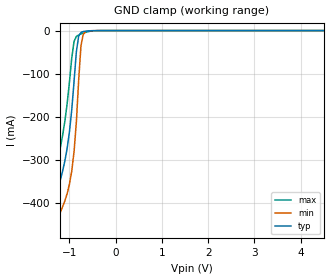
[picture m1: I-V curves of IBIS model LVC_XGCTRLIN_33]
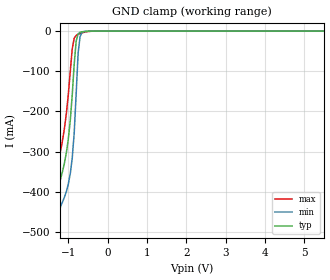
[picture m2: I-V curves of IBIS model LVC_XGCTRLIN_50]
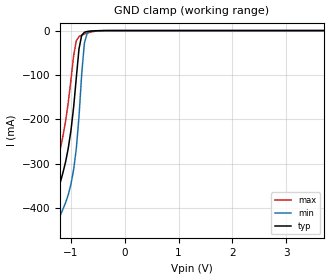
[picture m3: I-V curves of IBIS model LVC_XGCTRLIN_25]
| Philips Semiconductors Inc.
| Logic Products Group
| IBIS model of 74LVC2G125
| 3.3V DUAL BUS BUFFER/LINE DRIVER (3-STATE)
|[Packages]:
|[Package1]: SOT505-2 (TSSOP) 8-Pin Package ;
|[Package2]: SOT765 (VSSOP) 8-Pin Package ;
[IBIS Ver]   3.2
[File Name]   lvc2g125.ibs
[File Rev]   1.0
[Date]   25-Jul-2003
[Source]   File created from simulations by LPG
   Philips Semiconductors Nijmegen
[Notes]   V1.0   Ibis model.
| Revision History
| Version Date   Author/ Description
|   Editor
| 1.0   July   2003 RM   Initial Version
| Remarks:
| 1. The Power Clamp curves have been omitted since there is no power clamp
|   diode.
| 2. Non-monotonic sections below 0V in pulldown and pullup curves have been
|   removed (if any).
[Disclaimer]
   (C) Copyright 2003 Philips Semiconductors
   All rights reserved
   Philips Semiconductors warrants and represents that the IBIS model
   identified herein is owned by Philips Semiconductors (PHILIPS). The
   model provided is not warranted as fully representing all of the
   operating characteristics and specifications of the semiconductor
   products to which the model relates.  Moreover, unless there is a
   signed, written agreement to the contrary, this IBIS model is
   furnished on an "as is" basis without support or warranty of any
   kind, either expressed or implied, regarding the use thereof, and
   PHILIPS specifically disclaims all implied warranties of
   merchantability and fitness of the model for any purpose.
   PHILIPS does not assume any liability arising out of the application
   or use of this IBIS model including infringement of patents and
   copyrights, nor does PHILIPS convey any license under its patents and
   copyrights or the rights of others.
   PHILIPS provides IBIS models as a service to our customers. You and
   your company shall not distribute, convey, sell, or give these models
   to anyone else without receiving prior written permission from
   PHILIPS.
   PHILIPS reserves the right to make changes without notice to these
   IBIS models to improve reliability, function, or design.
   Please be aware that your receipt and subsequent use of the IBIS
   information provided shall serve as acceptance of the terms and
   conditions of this agreement.  If you do not accept these terms,
   you should return or destroy the IBIS models and any other
   accompanying information immediately.
|   Info for  SOT505-2 (TSSOP) 8-Pin Package
[Component]   74LVC2G125_1
[Manufacturer]   Philips Semiconductors Inc.
[Package]
|   typ   min   max
R_pkg   5.4457E-02   4.6527E-02   6.2827E-02
L_pkg   1.399E-09   1.251E-09   1.584E-09
C_pkg   9.08E-14   7.40E-14   1.08E-13
[Pin] signal_name   model_name   R_pin   L_pin   C_pin
   1   OE1#   lvc_xgctrlin 6.28E-02 1.584E-09  1.08E-13
   2   A1   lvc_xgin 4.72E-02 1.312E-09  7.50E-14
   3   Y2   lvc_xgtristn 4.65E-02 1.251E-09  7.40E-14
   4   GND   GND 6.15E-02 1.472E-09  1.07E-13
   5   A2   lvc_xgin 6.22E-02 1.484E-09  1.07E-13
   6   Y1   lvc_xgtristn 4.69E-02 1.256E-09  7.40E-14
   7   OE2#   lvc_xgctrlin 4.67E-02 1.304E-09  7.40E-14
   8   VCC   POWER 6.18E-02 1.527E-09  1.07E-13
|   Info for  SOT765 (VSSOP) 8-Pin Package
[Component]   74LVC2G125_2
[Manufacturer]   Philips Semiconductors Inc.
[Package]
|   typ   min   max
R_pkg   3.2883E-02   1.0000E-06   4.2432E-02
L_pkg   9.425E-10   1.000E-12   1.184E-09
C_pkg   8.64E-14   1.00E-15   1.19E-13
[Pin] signal_name   model_name   R_pin   L_pin   C_pin
   1   OE1#   lvc_xgctrlin 4.24E-02 1.145E-09  1.19E-13
   2   A1   lvc_xgin 3.40E-02 1.018E-09  8.30E-14
   3   Y2   lvc_xgtristn 3.40E-02 1.016E-09  8.40E-14
   4   GND   GND 4.24E-02  1.15E-09  1.19E-13
   5   A2   lvc_xgin 3.40E-02  9.89E-10  1.12E-13
   6   Y1   lvc_xgtristn 3.40E-02 1.037E-09  8.30E-14
   7   OE2#   lvc_xgctrlin 4.24E-02 1.184E-09  9.00E-14
   8   VCC   POWER 1.00E-06  1.00E-12  1.00E-15
[Model Selector]   lvc_xgctrlin
| Remark: If your software does not support the Model Selector
|   Please comment out the lines of the Model Selector, which
|   contain the name of the Model, except the one you want to use.
LVC_XGCTRLIN_33   3.3V-Vcc input model
LVC_XGCTRLIN_50   5.0V-Vcc input model
LVC_XGCTRLIN_25   2.5V-Vcc input model
LVC_XGCTRLIN_18   1.8V-Vcc input model
[Model Selector]   lvc_xgin
| Remark: If your software does not support the Model Selector
|   Please comment out the lines of the Model Selector, which
|   contain the name of the Model, except the one you want to use.
LVC_XGIN_33   3.3V-Vcc input model
LVC_XGIN_50   5.0V-Vcc input model
LVC_XGIN_25   2.5V-Vcc input model
LVC_XGIN_18   1.8V-Vcc input model
[Model Selector]   lvc_xgtristn
| Remark: If your software does not support the Model Selector
|   Please comment out the lines of the Model Selector, which
|   contain the name of the Model, except the one you want to use.
LVC_XGTRISTN_33   3.3V-Vcc tristate non-inverting output model
LVC_XGTRISTN_50   5.0V-Vcc tristate non-inverting output model
LVC_XGTRISTN_25   2.5V-Vcc tristate non-inverting output model
LVC_XGTRISTN_18   1.8V-Vcc tristate non-inverting output model
| Models and submodels in the file (12): LVC_XGCTRLIN_33 (Input), LVC_XGCTRLIN_50 (Input), LVC_XGCTRLIN_25 (Input), LVC_XGCTRLIN_18 (Input), LVC_XGIN_33 (Input), LVC_XGIN_50 (Input), LVC_XGIN_25 (Input), LVC_XGIN_18 (Input), LVC_XGTRISTN_33 (3-state), LVC_XGTRISTN_50 (3-state), LVC_XGTRISTN_25 (3-state), LVC_XGTRISTN_18 (3-state)
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|   Model LVC_XGCTRLIN_33
[Model]   LVC_XGCTRLIN_33
Model_type   Input
Vinl =   0.8V
Vinh =   2.0V
C_comp   2.96pF   2.12pF   3.91pF
[Model Spec]
| Note: The input and output voltage ratings may be exceeded if the input and
|   output current ratings are observed (please refer to the data sheet)
|   Subparameter   typ   min   max
| Thresholds
Vinh   2.0   2.0   2.0
Vinl   0.8   0.8   0.8
| Overshoot
S_overshoot_high   6.5   6.5   6.5   | Static overshoot
S_overshoot_low   -0.5   -0.5   -0.5
D_overshoot_high   7.2   7.2   7.2   | Dynamic overshoot
D_overshoot_low   -0.95   -0.9   -1.0
D_overshoot_time   3n   3n   3n
|Ambient temperature:   25   85   -40
[Temperature Range]   50   105   -10
[Voltage Range]   3.3V   3.0V   3.6V
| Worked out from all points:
|   GND clamp passes 1 mA (typ) near -0.61 V on its own axis
|Process Range   nominal   slow   fast
[GND_clamp]
| voltage   I(typ)   I(min)   I(max)
-5.5V     -4.562A    -4.619A    -4.506A
-1.45V    -549.4mA   -615.4mA   -482.8mA
-1.4V     -502.2mA   -568.5mA   -435.4mA
-1.35V    -455.9mA   -522.5mA   -388.7mA
-1.3V     -411.6mA   -478.9mA   -343.8mA
-1.1V     -304.2mA   -396.4mA   -212.1mA
-950mV    -185.2mA   -327mA     -64.69mA
-850mV    -49.8mA    -213.4mA   -13.79mA
-750mV    -4.324mA   -35.6mA    -7.884mA
-700mV    -2.27mA    -8.526mA   -5.841mA
-550mV    -593.6uA   -425.2uA   -1.597mA
5.5V      375.8pA    2.471nA    52.76pA
|   Model LVC_XGCTRLIN_50
[Model]   LVC_XGCTRLIN_50
Model_type   Input
Vinl =   1.5V
Vinh =   3.5V
C_comp   2.89pF   1.97pF   3.94pF
[Model Spec]
| Note: The input and output voltage ratings may be exceeded if the input and
|   output current ratings are observed (please refer to the data sheet)
|   Subparameter   typ   min   max
| Thresholds
Vinh   3.5   3.15   3.85
Vinl   1.5   1.35   1.65
| Overshoot
S_overshoot_high   6.5   6.5   6.5   | Static overshoot
S_overshoot_low   -0.5   -0.5   -0.5
D_overshoot_high   11.0   11.0   11.0   | Dynamic overshoot
D_overshoot_low   -0.95   -0.9   -1.0
D_overshoot_time   3n   3n   3n
|Ambient temperature:   25   85   -40
[Temperature Range]   50   105   -10
[Voltage Range]   5.0V   4.5V   5.5V
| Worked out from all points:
|   GND clamp passes 1 mA (typ) near -0.59 V on its own axis
|Process Range   nominal   slow   fast
[GND_clamp]
| voltage   I(typ)   I(min)   I(max)
-5.5V     -4.585A    -4.637A    -4.534A
-1.45V    -567.8mA   -628.4mA   -505.9mA
-1.4V     -520.6mA   -581.5mA   -458.5mA
-1.3V     -430.1mA   -491.9mA   -367mA
-1.2V     -369.6mA   -437.9mA   -299.9mA
-1.05V    -303mA     -399.7mA   -205.6mA
-950mV    -222.3mA   -354.8mA   -100.4mA
-850mV    -82.04mA   -253.9mA   -17.37mA
-800mV    -24.94mA   -156mA     -10.72mA
-750mV    -6.792mA   -54.58mA   -8.095mA
-700mV    -2.837mA   -13.44mA   -6.14mA
5.5V      1.794nA    5.479nA    963.8pA
|   Model LVC_XGCTRLIN_25
[Model]   LVC_XGCTRLIN_25
Model_type   Input
Vinl =   0.7V
Vinh =   1.7V
C_comp   3.01pF   2.23pF   3.90pF
[Model Spec]
| Note: The input and output voltage ratings may be exceeded if the input and
|   output current ratings are observed (please refer to the data sheet)
|   Subparameter   typ   min   max
| Thresholds
Vinh   1.7   1.7   1.7
Vinl   0.7   0.7   0.7
| Overshoot
S_overshoot_high   6.5   6.5   6.5   | Static overshoot
S_overshoot_low   -0.5   -0.5   -0.5
D_overshoot_high   7.2   7.2   7.2   | Dynamic overshoot
D_overshoot_low   -0.95   -0.9   -1.0
D_overshoot_time   3n   3n   3n
|Ambient temperature:   25   85   -40
[Temperature Range]   30   90   -35
[Voltage Range]   2.5V   2.3V   2.7V
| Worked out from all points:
|   GND clamp passes 1 mA (typ) near -0.61 V on its own axis
|Process Range   nominal   slow   fast
[GND_clamp]
| voltage   I(typ)   I(min)   I(max)
-5.5V     -4.553A    -4.61A     -4.497A
-1.45V    -543.2mA   -609mA     -477mA
-1.4V     -496.1mA   -562.1mA   -429.6mA
-1.35V    -449.7mA   -516.1mA   -382.9mA
-1.25V    -367.8mA   -436.8mA   -298.4mA
-1.1V     -295.9mA   -387.6mA   -204.4mA
-950mV    -173.1mA   -313.3mA   -57.16mA
-850mV    -41.37mA   -194.3mA   -13.46mA
-750mV    -3.847mA   -28.54mA   -7.836mA
-700mV    -2.146mA   -6.789mA   -5.759mA
-550mV    -554.2uA   -385.7uA   -1.497mA
5.5V      211.8pA    1.646nA    21.33pA
